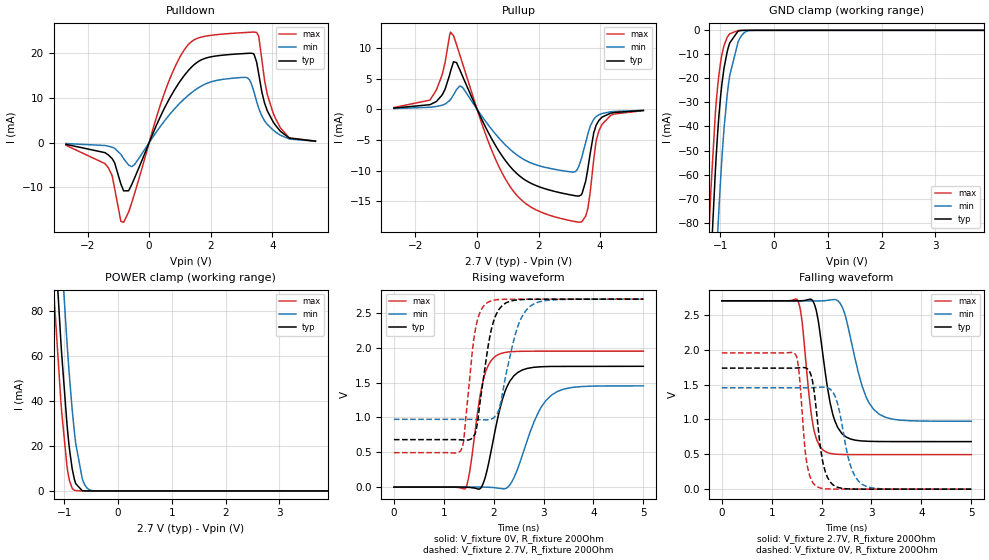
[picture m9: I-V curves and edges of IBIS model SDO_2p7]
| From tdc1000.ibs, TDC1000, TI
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|   Model
[Model]   SDO_2p7
Model_type   I/O
Polarity   Non-Inverting
Enable   Active-Low
Vinl = 0.81
Vinh = 1.89
Vmeas = 1.35
Vref = 0
Cref = 1pF
Rref = 100000
|   typ   min   max
C_comp   0.670pF   0.613pF   0.704pF
[Voltage Range]   2.7   2.699   2.701
[Temperature Range]   27   125   -40
[Pullup Reference]   2.7   2.699   2.701
[Pulldown Reference]   0   0   0
[Power Clamp Reference]   2.7   2.699   2.701
[GND Clamp Reference]   0   0   0
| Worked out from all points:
|   slope of the pulldown table from 0 to 0.405 V, typ, clamps not added: 63.4 ohm
|   slope of the pullup table from 0 to 0.405 V, typ, clamps not added: 97 ohm
|   GND clamp passes 1 mA (typ) near -0.69 V on its own axis
|   POWER clamp passes 1 mA (typ) near -0.70 V on its own axis
|   falling waveform, V_fixture 2.7V, R_fixture 200Ohm: 20-80 % time 263ps typ, 372ps min, 195ps max; typ from 2.7 V to 0.682 V
|   rising waveform, V_fixture 0V, R_fixture 200Ohm: 20-80 % time 335ps typ, 473ps min, 246ps max; typ from 0 V to 1.74 V
|   rising waveform, V_fixture 2.7V, R_fixture 200Ohm: 20-80 % time 261ps typ, 338ps min, 198ps max; typ from 0.682 V to 2.7 V
|   falling waveform, V_fixture 0V, R_fixture 200Ohm: 20-80 % time 186ps typ, 261ps min, 138ps max; typ from 1.74 V to 0 V
[Pulldown]
|   Voltage   I(typ)   I(min)   I(max)
-2.7V     -382.3uA   -200.2uA   -596.1uA
-1.339V   -2.67mA    -764.1uA   -5.486mA
-828.9mV  -10.75mA   -3.568mA   -17.74mA
-488.7mV  -8.133mA   -4.989mA   -11.67mA
450.9mV   7.046mA    4.42mA     10.17mA
1.147V    15.03mA    9.796mA    20.77mA
2.508V    19.58mA    14.22mA    24.27mA
3.391V    19.79mA    11.62mA    24.65mA
3.561V    15.2mA     7.596mA    23.59mA
3.748V    8.822mA    4.876mA    13.88mA
4.25V     2.622mA    1.705mA    3.419mA
5.4V      324.5uA    299uA      351.4uA
[GND Clamp]
|   Voltage   I(typ)   I(min)   I(max)
-2.7V     -1.032A    -1.081A    -997.1mA
-1.339V   -187.4mA   -237.8mA   -155.3mA
-1.193V   -107.7mA   -157mA     -77.08mA
-1.169V   -95.4mA    -144.2mA   -65.54mA
-1.088V   -58.33mA   -103.8mA   -34.4mA
-1.048V   -43.29mA   -85.27mA   -23.7mA
-990.9mV  -27.43mA   -61.95mA   -13.28mA
-934.2mV  -16.76mA   -42.84mA   -6.897mA
-820.8mV  -5.226mA   -18.67mA   -1.439mA
-666.9mV  -329uA     -4.846mA   -100.2uA
-464.4mV  -1.391uA   -139.9uA   -332.9nA
5.4V      0A         0A         0A
[Pullup]
|   Voltage   I(typ)   I(min)   I(max)
-2.7V     196.6uA    122.5uA    282.3uA
-1.526V   759.6uA    334.4uA    1.538mA
-1.145V   2.267mA    649.2uA    5.464mA
-861.3mV  6.208mA    1.595mA    12.6mA
-480.6mV  5.514mA    3.605mA    7.617mA
369.9mV   -3.845mA   -2.604mA   -5.343mA
1.091V    -9.452mA   -6.63mA    -12.75mA
3.31V     -14.17mA   -9.24mA    -18.44mA
3.594V    -9.837mA   -4.108mA   -16.29mA
3.861V    -2.688mA   -1.23mA    -5.385mA
4.055V    -1.294mA   -696.5uA   -2.484mA
5.4V      -193.9uA   -164.1uA   -218.9uA
[POWER Clamp]
|   Voltage   I(typ)   I(min)   I(max)
-2.7V     892.6mA    954.2mA    841.5mA
-1.202V   122.2mA    169.6mA    90.73mA
-1.064V   66.49mA    109.6mA    39.99mA
-1.048V   60.6mA     103mA      34.93mA
-950.4mV  29.81mA    66.2mA     11.12mA
-926.1mV  23.65mA    57.94mA    7.305mA
-853.2mV  9.845mA    36.13mA    1.163mA
-812.7mV  5.182mA    26.28mA    304.9uA
-666.9mV  107.4uA    5.507mA    7.619uA
-585.9mV  7.429uA    1.557mA    969.7nA
-480.6mV  286.4nA    155.5uA    23.31nA
5.4V      0A         0A         0A
[Ramp]
R_load = 200
|   typ   min   max
dV/dt_r   1.04111/3.35366e-10   0.872513/4.72546e-10   1.17165/2.46269e-10
dV/dt_f   1.21089/2.63073e-10   1.03539/3.72494e-10   1.32371/1.94852e-10
[Falling Waveform]
V_fixture = 2.7V
V_fixture_min = 2.699V
V_fixture_max = 2.701V
R_fixture = 200Ohm
C_fixture = 0F
|   Time   V(typ)   V(min)   V(max)
0s        2.7V       2.699V     2.701V
1.516ns   2.699V     2.699V     2.713V
1.607ns   2.701V     2.699V     2.414V
1.836ns   2.684V     2.698V     885.8mV
2.086ns   1.606V     2.703V     533.5mV
2.224ns   1.074V     2.716V     506.6mV
2.405ns   797.9mV    2.623V     497.5mV
2.809ns   690.9mV    1.483V     494.9mV
3.16ns    683mV      1.072V     494.8mV
5ns       681.9mV    973.4mV    494.8mV
[Rising Waveform]
V_fixture = 0V
V_fixture_min = 0V
V_fixture_max = 0V
R_fixture = 200Ohm
C_fixture = 0F
|   Time   V(typ)   V(min)   V(max)
0s        -51.19nV   162.7nV    1.285uV
1.429ns   -591.8uV   445.2uV    -23.26mV
1.516ns   -4.745mV   472.4uV    211.5mV
1.778ns   32.85mV    259.3uV    1.494V
1.905ns   366.2mV    -2.26mV    1.767V
2.086ns   1.009V     -14.75mV   1.902V
2.405ns   1.599V     133mV      1.947V
2.893ns   1.726V     1.072V     1.953V
3.16ns    1.733V     1.322V     1.953V
5ns       1.735V     1.454V     1.953V
[Rising Waveform]
V_fixture = 2.7V
V_fixture_min = 2.699V
V_fixture_max = 2.701V
R_fixture = 200Ohm
C_fixture = 0F
|   Time   V(typ)   V(min)   V(max)
0s        681.9mV    973.3mV    494.8mV
1.341ns   679.1mV    973.5mV    525.8mV
1.395ns   677.3mV    973.5mV    649.9mV
1.628ns   767.3mV    971.8mV    2.244V
1.868ns   1.927V     965.8mV    2.647V
1.985ns   2.353V     988.5mV    2.681V
2.115ns   2.562V     1.143V     2.694V
2.45ns    2.687V     2.233V     2.699V
2.733ns   2.698V     2.598V     2.699V
5ns       2.7V       2.699V     2.701V
[Falling Waveform]
|Gnd
V_fixture = 0V
V_fixture_min = 0V
V_fixture_max = 0V
R_fixture = 200Ohm
C_fixture = 0F
|   Time   V(typ)   V(min)   V(max)
0s        1.735V     1.454V     1.953V
1.479ns   1.736V     1.454V     1.928V
1.535ns   1.738V     1.454V     1.755V
1.712ns   1.726V     1.454V     335.4mV
1.905ns   1.057V     1.458V     36.85mV
2.015ns   423.2mV    1.462V     10.66mV
2.17ns    105.2mV    1.433V     2.52mV
2.61ns    2.174mV    272.6mV    715.4uV
2.809ns   659.1uV    71.37mV    655.6uV
5ns       -54.24nV   924.6nV    -1.29uV
